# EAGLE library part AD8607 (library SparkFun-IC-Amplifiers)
Micropower Low-noise Rail to Rail OP-AMP Datasheet SparkFun Products () Currently in prototype (unknown project)
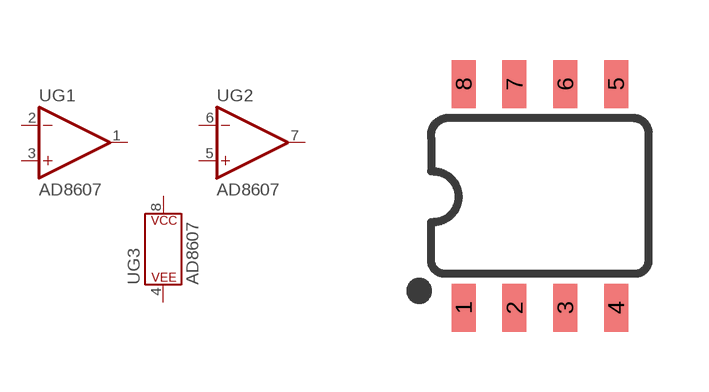
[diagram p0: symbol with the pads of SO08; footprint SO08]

Designator prefix U; gates G1=OP-AMP G2=OP-AMP G3=POWER_CONSORT

## AD8607 (PROD_ID: IC-13133; VALUE: AD8607)  [SO08]
1  G1:OUT  out
2  G1:-IN  in
3  G1:+IN  in
4  G3:P$V-
5  G2:+IN  in
6  G2:-IN  in
7  G2:OUT  out
8  G3:P$V+

## Footprint SO08 (pad centres in mm)
SOIC, 0.15 inch width
smd 0.6 x 1.2: 1 -1.905,-2.8; 2 -0.635,-2.8; 3 0.635,-2.8; 4 1.905,-2.8; 5 1.905,2.8; 6 0.635,2.8; 7 -0.635,2.8; 8 -1.905,2.8

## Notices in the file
Licensing: Creative Commons ShareAlike 4.0 International - https://creativecommons.org/licenses/by-sa/4.0
